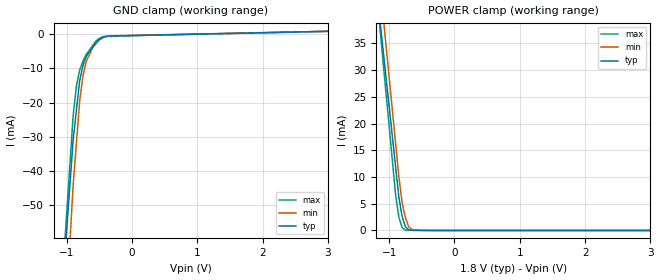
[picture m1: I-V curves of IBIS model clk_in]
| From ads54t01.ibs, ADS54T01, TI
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[Model] clk_in
Model_type Input
Vinl = 1.12500V
Vinh = 1.37500V
C_comp 1.11000pF 1.03000pF 1.19000pF
| variable typ   min   max
[Voltage Range] 1.80000V 1.65000V 1.95000V
[POWER Clamp Reference] 1.80000V 1.65000V 1.95000V
[GND Clamp Reference] 0.00000V 0.00000V 0.00000V
[Temperature Range]   25   85   -40
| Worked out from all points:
|   GND clamp passes 1 mA (typ) near -0.46 V on its own axis
|   POWER clamp passes 1 mA (typ) near -0.76 V on its own axis
[GND Clamp]
-1.8V     -272.1mA   -350.5mA   -285mA
-900mV    -31.01mA   -44.28mA   -23.91mA
-850mV    -22.31mA   -31.92mA   -15.15mA
-800mV    -13.6mA    -19.57mA   -10.48mA
-750mV    -9.108mA   -12.21mA   -7.854mA
-700mV    -6.486mA   -7.922mA   -5.891mA
-600mV    -3.678mA   -3.87mA    -3.255mA
-550mV    -2.274mA   -2.771mA   -1.937mA
-500mV    -1.434mA   -1.672mA   -1.171mA
-400mV    -604.3uA   -655.7uA   -566.4uA
-175mV    -420.1uA   -360.8uA   -434.6uA
3.6V      1.167mA    1.154mA    1.158mA
[POWER Clamp]
-1.8V     114.7mA    128.8mA    123.8mA
-1.05V    29.03mA    35.03mA    26.14mA
-900mV    11.9mA     16.29mA    6.612mA
-850mV    6.185mA    10.04mA    2.484mA
-800mV    2.59mA     5.154mA    519.3uA
-750mV    699uA      2.372mA    71.89uA
-700mV    131.6uA    705.1uA    63.9uA
-650mV    19.66uA    158.6uA    55.91uA
-600mV    16.63uA    31uA       47.92uA
3.6V      0A         0A         0A
